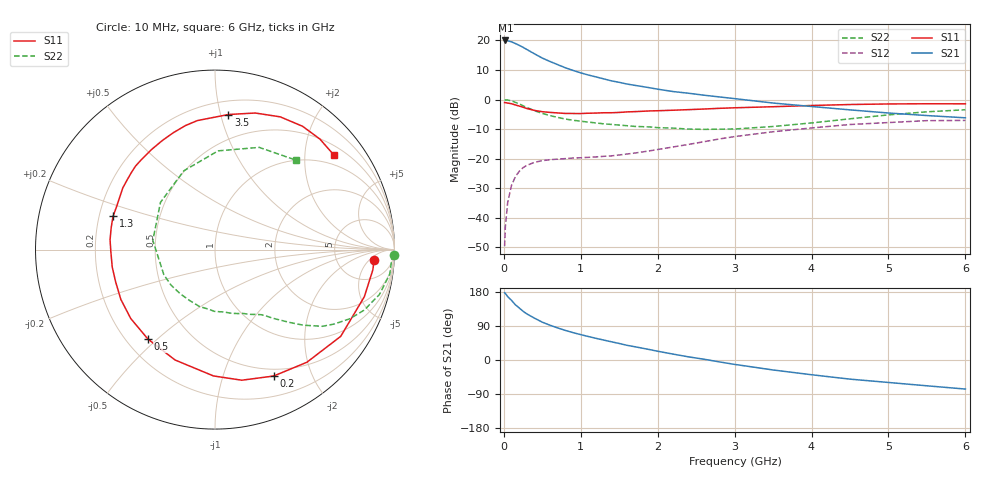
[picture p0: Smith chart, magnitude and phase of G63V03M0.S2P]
! SIEMENS Small Signal Semiconductors
! BFG193
! Si NPN RF Bipolar Junction Transistor in SOT223
! VCE = 3 V  IC = 3 mA
! Common Emitter S-Parameters:  August  1996
# GHz  S  MA  R  50
!  f  S11  S21  S12  S22
! GHz  MAG  ANG  MAG  ANG  MAG  ANG  MAG  ANG
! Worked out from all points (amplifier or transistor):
!   36 points, 10 MHz to 6 GHz, reference 50 ohm
!   highest |S21| = 20.0 dB at 20 MHz (marker M1)
!   |S21| within 3 dB of that: start of sweep to 295.1 MHz
!   unconditionally stable (mu >= 1): 1.273 GHz to 2.61 GHz
!   at 250 MHz: K = 0.23, MSG = 20.4 dB, |S12| = -23.0 dB
!   at 1.4 GHz: K = 1.08, MAG = 10.9 dB, |S12| = -19.1 dB
!   at 6 GHz: K = 0.93, MSG = 0.4 dB, |S12| = -7.1 dB
!   S11 on the Smith chart (normalised r, x): 10 MHz: 13, -7; 200 MHz: 0.42, -1.48; 500 MHz: 0.29, -0.47; 1.3 GHz: 0.26, +0.15; 3.5 GHz: 0.30, +1.06; 6 GHz: 0.73, +2.71
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0.01  0.8881 -3.7  9.973 177.4  0.0033 90.8  0.9955 -1.6
0.02  0.8867 -7.3  10.01 175.8  0.0071 88.1  0.986 -3.2
0.05  0.8725 -17.5  9.866 167.3  0.0181 79.7  0.9832 -8.0
0.1  0.851 -34.6  9.485 157.4  0.0353 72.2  0.9494 -15.3
0.15  0.81 -50.8  8.87 145.7  0.0494 62.7  0.8968 -22.1
0.2  0.7765 -65.1  8.281 137.3  0.061 57.0  0.8448 -27.1
0.25  0.7429 -78.4  7.661 128.7  0.0704 50.8  0.7853 -31.8
0.3  0.7039 -90.7  7.024 121.5  0.0771 46.1  0.7359 -35.5
0.4  0.6541 -109.9  5.93 110.2  0.0867 39.1  0.6471 -40.6
0.5  0.623 -126.8  5.031 99.8  0.0924 33.7  0.5826 -44.2
0.6  0.6065 -140.7  4.411 91.8  0.0961 30.7  0.5355 -47.2
0.7  0.5935 -152.1  3.897 84.6  0.0981 28.9  0.4986 -50.0
0.9  0.5808 -170.3  3.112 72.2  0.1023 26.7  0.4465 -54.4
1.1  0.5872 174.7  2.599 61.9  0.1052 27.0  0.4148 -60.5
1.3  0.5977 161.9  2.235 52.5  0.1095 28.2  0.3878 -66.4
1.6  0.6179 146.3  1.832 38.8  0.1197 30.5  0.361 -77.7
2.2  0.6599 122.6  1.367 15.6  0.1577 32.0  0.3287 -105.3
2.8  0.7104 103.4  1.109 -4.9  0.2151 26.4  0.315 -141.0
3.5  0.7564 84.3  0.873 -26.3  0.2854 12.2  0.35 171.6
4.5  0.8242 63.8  0.669 -50.5  0.3782 -10.0  0.4721 111.6
5.5  0.849 46.5  0.536 -68.1  0.4396 -37.3  0.6205 66.6
6  0.8466 38.3  0.491 -76.7  0.4433 -52.4  0.6724 47.8
